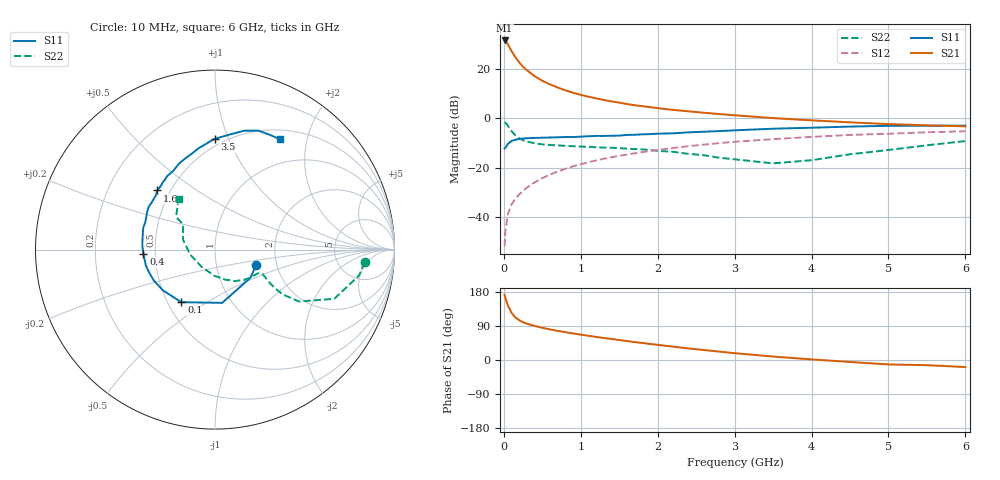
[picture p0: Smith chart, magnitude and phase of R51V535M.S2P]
! SIEMENS Small Signal Semiconductors
! BFR183
! Si NPN RF Bipolar Junction Transistor in SOT23
! VCE = 1.5 V  IC = 35 mA
! Common Emitter S-Parameters:  May  1996
# GHz  S  MA  R  50
!  f  S11  S21  S12  S22
! GHz  MAG  ANG  MAG  ANG  MAG  ANG  MAG  ANG
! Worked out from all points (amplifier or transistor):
!   36 points, 10 MHz to 6 GHz, reference 50 ohm
!   highest |S21| = 31.8 dB at 10 MHz (marker M1)
!   |S21| within 3 dB of that: start of sweep to 77.15 MHz
!   unconditionally stable (mu >= 1): start of sweep to 16.54 MHz; 225.2 MHz to 2.944 GHz
!   at 250 MHz: K = 1.03, MAG = 24.2 dB, |S12| = -29.5 dB
!   at 1.4 GHz: K = 1.12, MAG = 9.3 dB, |S12| = -15.8 dB
!   at 6 GHz: K = 0.99, MSG = 1.0 dB, |S12| = -5.2 dB
!   S11 on the Smith chart (normalised r, x): 10 MHz: 1.56, -0.29; 100 MHz: 0.59, -0.39; 400 MHz: 0.43, -0.02; 1.6 GHz: 0.42, +0.36; 3.5 GHz: 0.45, +0.89; 6 GHz: 0.63, +1.57
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0.01  0.2448 -21.0  38.69 172.1  0.0025 77.1  0.836 -4.8
0.02  0.2519 -38.7  37.9 164.3  0.0049 78.3  0.8162 -10.1
0.05  0.2994 -82.3  32.8 145.0  0.011 70.8  0.7191 -22.4
0.1  0.3479 -122.6  23.54 124.4  0.0177 65.6  0.5504 -31.7
0.15  0.3688 -142.1  17.57 112.3  0.0231 66.7  0.4519 -33.5
0.2  0.382 -153.4  13.8 104.9  0.0283 69.2  0.3945 -32.7
0.25  0.3898 -161.8  11.25 99.6  0.0335 70.1  0.3576 -31.4
0.3  0.3953 -167.4  9.559 95.8  0.039 71.0  0.3376 -30.1
0.4  0.3992 -176.5  7.279 90.0  0.0499 72.7  0.3113 -28.2
0.5  0.4052 177.3  5.849 84.9  0.0605 73.0  0.2956 -27.1
0.6  0.4083 171.6  4.927 80.8  0.072 72.8  0.2876 -27.2
0.7  0.4128 166.7  4.26 76.8  0.0828 72.5  0.2821 -27.8
0.9  0.4176 158.4  3.329 70.1  0.1059 71.1  0.2713 -29.4
1.1  0.4334 150.6  2.767 63.9  0.1284 69.2  0.2634 -32.7
1.3  0.4394 143.3  2.371 58.1  0.151 67.1  0.2547 -35.7
1.6  0.4608 134.3  1.964 50.0  0.1838 63.7  0.2417 -42.1
2.2  0.4969 117.8  1.491 35.2  0.25 55.9  0.2087 -57.4
2.8  0.552 103.1  1.227 22.2  0.3138 47.5  0.1581 -80.3
3.5  0.617 90.2  1.014 9.1  0.3787 37.0  0.1214 -128.4
4.5  0.6818 76.3  0.833 -5.2  0.4609 22.9  0.1862 162.9
5.5  0.7086 64.5  0.724 -13.7  0.5219 10.8  0.2835 139.9
6  0.7138 59.3  0.69 -18.6  0.5481 3.1  0.3454 126.0
